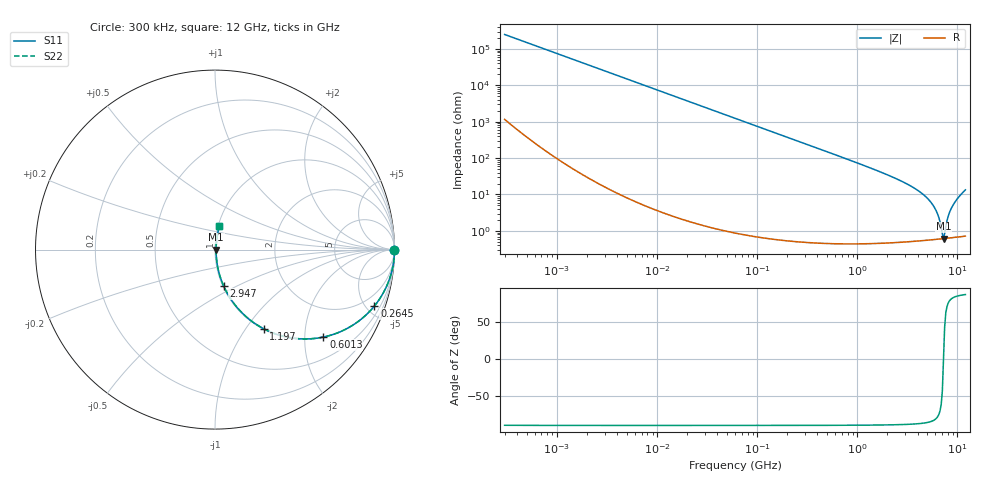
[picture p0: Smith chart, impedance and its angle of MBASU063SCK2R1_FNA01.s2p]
! MBASU063SCK2R1_FNA01  S-PARAMETER MODEL  ( General Type )
! Model Generated by TAIYO YUDEN Corporation (http://www.ty-top.com)
! Version 1.0
! TAIYO YUDEN Control No. 130801
! Copyright(c) 2013 TAIYO YUDEN CO.,LTD. All Rights Reserved.
! Product Description (link to TY-COMPAS)
! https://ds.yuden.co.jp/TYCOMPAS/or/detail?pn=MBASU063SCK2R1CFNA01&u=M
! Products Name : Multilayer Ceramic Capacitors
! Characteristics :
!  Capacitance : 2.1 pF , Rated Voltage : 50V , TCC : CK / C0K
!  Case Size : 0.6 x 0.3 / 0.024 x 0.012 [mm/inch] , Thickness : 0.3 / 0.012 [mm/inch]
!  (Conditions: Temperature = 25 degC , DC Bias Current/Voltage = 0A / 0V)
! External Node Assignments :
!  1  o---| |---o  2
! GND o---------o GND
! Frequency Range : 0.3MHz  -  12000MHz  [ 401 STEP ]
# MHz S RI R 50
! Freq[MHz].  S11 Real  S11 Imag  S21 Real  S21 Imag  S12 Real  S12 Imag  S22 Real  S22 Imag
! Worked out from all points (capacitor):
!   401 points, 300 kHz to 12 GHz, reference 50 ohm
!   read as one part in series: C = 2.12 pF near 316.3 kHz
!   lowest |Z| = 612 mohm at 7.254 GHz (marker M1)
!   series resonance near 7.259 GHz, so ESL is about 230 pH
!   S11 on the Smith chart (normalised r, x): 300 kHz: open; 264.5 MHz: 1.01, -5.66; 601.3 MHz: 1.01, -2.47; 1.197 GHz: 1.01, -1.22; 2.947 GHz: 1.01, -0.42; 12 GHz: 1.01, +0.27
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0.3  1 -0.0004  2.02e-06 0.0004  2.02e-06 0.0004  1 -0.0004
1.769972  1 -0.00236  7.6e-06 0.00236  7.6e-06 0.00236  1 -0.00236
10.44266  0.9998 -0.0139  0.000201 0.0139  0.000201 0.0139  0.9998 -0.0139
60  0.9936 -0.0796  0.00643 0.0796  0.00643 0.0796  0.9936 -0.0796
129.3602  0.9709 -0.1677  0.0291 0.1677  0.0291 0.1677  0.9709 -0.1677
264.5085  0.8884 -0.314  0.1116 0.314  0.1116 0.314  0.8884 -0.314
353.9943  0.8162 -0.3862  0.1838 0.3862  0.1838 0.3862  0.8162 -0.3862
601.3112  0.6045 -0.4872  0.3955 0.4872  0.3955 0.4872  0.6045 -0.4872
1197.383  0.2717 -0.4412  0.7283 0.4412  0.7283 0.4412  0.2717 -0.4412
2088.533  0.101 -0.2944  0.899 0.2944  0.899 0.2944  0.101 -0.2944
2947.191  0.0474 -0.2012  0.9526 0.2012  0.9526 0.2012  0.0474 -0.2012
4270.516  0.0181 -0.1121  0.9819 0.1121  0.9819 0.1121  0.0181 -0.1121
5420.343  0.00929 -0.0603  0.9907 0.0603  0.9907 0.0603  0.00929 -0.0603
6188.031  0.0069 -0.0328  0.9931 0.0328  0.9931 0.0328  0.0069 -0.0328
6524.734  0.00638 -0.0219  0.9936 0.0219  0.9936 0.0219  0.00638 -0.0219
6879.757  0.00611 -0.011  0.9939 0.011  0.9939 0.011  0.00611 -0.011
7254.098  0.00608 -0.000139  0.9939 0.000139  0.9939 0.000139  0.00608 -0.000139
7448.838  0.00616 0.00576  0.9938 -0.00576  0.9938 -0.00576  0.00616 0.00576
8281.503  0.00722 0.0299  0.9928 -0.0299  0.9928 -0.0299  0.00722 0.0299
8966.534  0.00881 0.0481  0.9912 -0.0481  0.9912 -0.0481  0.00881 0.0481
10236.47  0.0135 0.0816  0.9865 -0.0816  0.9865 -0.0816  0.0135 0.0816
12000  0.0244 0.1297  0.9756 -0.1297  0.9756 -0.1297  0.0244 0.1297
